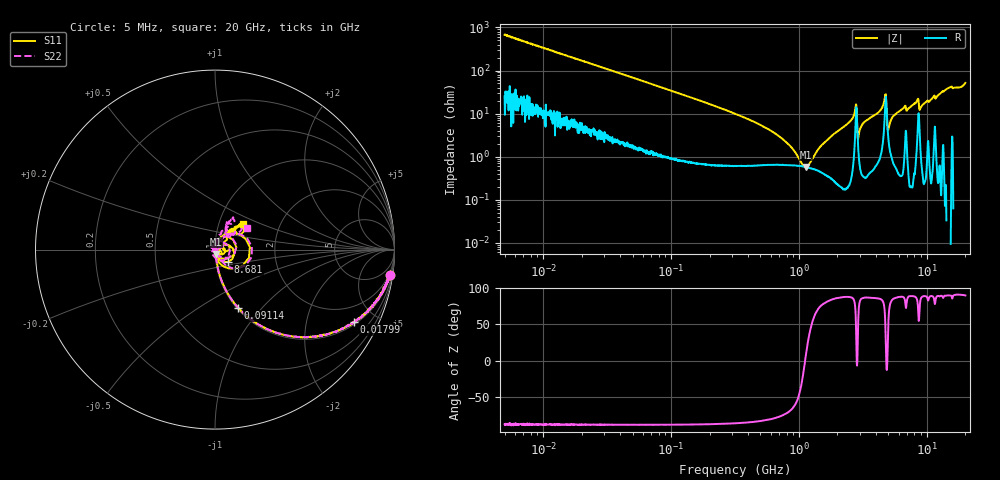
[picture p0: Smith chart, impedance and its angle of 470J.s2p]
!Keysight Technologies,P5008B,MY61100088,A.16.20.02
!Date: Wednesday, November 08, 2023 15:07:22
!Correction: S11(C  2-Port  )
!S21(C  2-Port  )
!S12(C  2-Port  )
!S22(C  2-Port  )
!S2P File: Measurements: S11, S21, S12, S22:Log Frequency Sweep
# Hz S  dB  R 50
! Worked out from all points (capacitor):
!   1601 points, 5 MHz to 20 GHz, reference 50 ohm
!   read as one part in series: C = 47.3 pF near 5.212 MHz
!   lowest |Z| = 570 mohm at 1.126 GHz (marker M1)
!   series resonance near 1.116 GHz, so ESL is about 430 pH
!   S11 on the Smith chart (normalised r, x): 5 MHz: 1, -13; 17.99 MHz: 1.12, -3.77; 91.14 MHz: 1.02, -0.75; 8.681 GHz: 1.14, -0.16; 20 GHz: 1.31, +0.39
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5000000  -0.14 -8.4  -16.74 79.5  -16.74 79.5  -0.14 -8.3
1.799028e7  -1.18 -27.5  -6.71 60.7  -6.71 60.7  -1.18 -27.5
1.995555e7  -1.37 -30.0  -6.02 58.6  -6.02 58.6  -1.37 -30.0
7.964482e7  -8.12 -65.6  -0.82 23.0  -0.82 23.0  -8.13 -65.7
9.113622e7  -9.13 -68.2  -0.65 20.3  -0.65 20.3  -9.14 -68.2
3.162278e8  -19.62 -81.1  -0.10 5.4  -0.10 5.4  -19.86 -81.7
1.12607e9  -32.28 -78.3  -0.08 -1.1  -0.08 -1.1  -39.24 -91.3
1.2621e9  -33.50 -80.3  -0.08 -1.6  -0.08 -1.6  -42.64 -101.2
1.451706e9  -37.00 -86.3  -0.08 -2.2  -0.08 -2.2  -53.38 -175.4
1.881234e9  -48.41 -176.5  -0.08 -3.6  -0.09 -3.6  -39.00 112.5
2.732345e9  -23.34 69.2  -0.27 -8.5  -0.27 -8.5  -23.79 70.5
2.848039e9  -24.15 -52.3  -0.56 -2.2  -0.56 -2.1  -23.27 -42.2
2.98406e9  -46.57 -167.1  -0.11 -4.9  -0.12 -4.9  -40.86 -76.7
3.110411e9  -37.36 118.8  -0.09 -5.8  -0.09 -5.8  -49.92 31.3
4.684567e9  -16.99 40.9  -0.80 -16.0  -0.80 -16.0  -16.64 38.0
5.037181e9  -26.86 -80.9  -0.18 -7.5  -0.18 -7.5  -25.89 -61.4
5.915309e9  -43.14 -16.3  -0.03 -12.2  -0.04 -12.2  -44.82 55.6
6.698975e9  -29.04 21.0  -0.12 -15.3  -0.12 -15.3  -30.45 83.2
8.681059e9  -20.03 -43.8  -0.67 -16.7  -0.68 -16.7  -22.20 -49.9
1.019442e10  -27.63 -25.0  -0.18 -23.0  -0.18 -22.9  -36.89 19.9
1.362808e10  -16.99 46.3  -0.09 -31.2  -0.09 -31.2  -17.14 64.3
2e10  -13.47 42.3  -0.24 -52.5  -0.24 -52.5  -13.38 34.6
